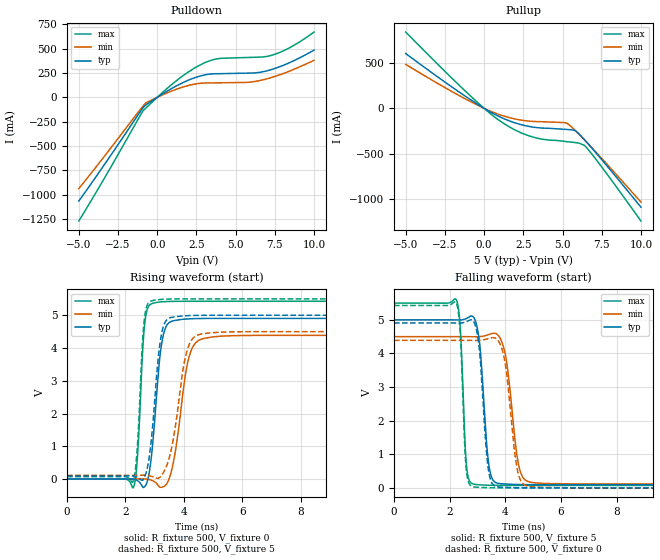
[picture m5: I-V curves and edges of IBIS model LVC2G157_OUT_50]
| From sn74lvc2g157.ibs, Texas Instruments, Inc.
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[Model]   LVC2G157_OUT_50
Model_type  Output
Vref =   0
Rref =   500
Cref =   50p
Vmeas =   2.5
| variable   typ   min   max
C_comp   8.88pF   5.48pF   12.17pF
| C_pullup   9.50pF   5.48pF   12.17pF
| C_pulldown   8.25pF   6.13pF   11.11pF
[Temperature Range]   40   100   -40
| Ambient temperature   25   85   -40
[Voltage range]   5   4.5   5.5
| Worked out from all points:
|   slope of the pulldown table from 0 to 0.75 V, typ, clamps not added: 9.95 ohm
|   slope of the pullup table from 0 to 0.75 V, typ, clamps not added: 10.3 ohm
|   rising waveform, R_fixture 500, V_fixture 0: 20-80 % time 283ps typ, 407ps min, 181ps max; typ from 0 V to 4.9 V
|   falling waveform, R_fixture 500, V_fixture 5: 20-80 % time 245ps typ, 345ps min, 159ps max; typ from 5 V to 0.093 V
|   rising waveform, R_fixture 500, V_fixture 5: 20-80 % time 293ps typ, 440ps min, 182ps max; typ from 0.093 V to 5 V
|   falling waveform, R_fixture 500, V_fixture 0: 20-80 % time 242ps typ, 334ps min, 155ps max; typ from 4.91 V to 0 V
[Pulldown]
| LVC2G157_OUT_50
|   Voltage   I(typ)   I(min)   I(max)
-5V       -1.064A    -937.1mA   -1.27A
-3.355V   -687.5mA   -602.1mA   -826.3mA
-925mV    -111.5mA   -92.93mA   -143.7mA
-620mV    -65.83mA   -48.5mA    -93.56mA
1.13V     109.8mA    78.31mA    159.2mA
2.415V    202.9mA    136.7mA    304.4mA
3.52V     241.4mA    148.6mA    384.4mA
5.67V     248.7mA    153.7mA    409.3mA
6.55V     257.8mA    173.2mA    413.7mA
7.245V    283.9mA    202mA      430mA
8.045V    329.6mA    245.5mA    478mA
10V       485.6mA    380.4mA    671.3mA
[Pullup]
| LVC2G157_OUT_50
|   Voltage   I(typ)   I(min)   I(max)
-5V       604.5mA    484.9mA    841.8mA
-1.075V   119.7mA    93.33mA    170.1mA
205mV     -21.37mA   -16.3mA    -30.84mA
1.085V    -100.6mA   -75.34mA   -147.2mA
2.055V    -164.7mA   -120mA     -245.4mA
3.025V    -204.3mA   -143.2mA   -312mA
3.86V     -218.8mA   -148.7mA   -344.2mA
5.29V     -233.1mA   -166mA     -367.5mA
5.825V    -248.5mA   -246.2mA   -378.1mA
6.49V     -363.8mA   -364.1mA   -425.3mA
7.725V    -612.1mA   -595.3mA   -698.9mA
10V       -1.09A     -1.034A    -1.243A
[Ramp]
| LVC2G157_OUT_50
| variable   typ   min   max
dV/dt_r   3.10/3.12E-10   2.78/4.40E-10   3.42/1.94E-10
dV/dt_f   3.01/2.60E-10   2.69/3.61E-10   3.33/1.65E-10
R_load = 500
[Rising Waveform]
| LVC2G157_OUT_50
R_fixture =   500
C_fixture =   0
L_fixture =   0
V_fixture =   0
V_fixture_min = 0
V_fixture_max = 0
|   Time   V(typ)   V(min)   V(max)
0s        187.4pV    4.471nV    591.1pV
2.275ns   -2.539mV   258.5uV    -248.9mV
2.41ns    -46.69mV   1.381mV    678.3mV
2.66ns    -227.1mV   4.361mV    4.753V
2.965ns   1.407V     -67.03mV   5.372V
3.18ns    3.746V     -247.6mV   5.404V
3.385ns   4.647V     -175.4mV   5.418V
4.175ns   4.89V      3.718V     5.426V
4.715ns   4.902V     4.299V     5.427V
24.99ns   4.904V     4.387V     5.427V
[Falling Waveform]
| LVC2G157_OUT_50
R_fixture =   500
C_fixture =   0
L_fixture =   0
V_fixture =   5
V_fixture_min = 4.5
V_fixture_max = 5.5
|   Time   V(typ)   V(min)   V(max)
0s        5V         4.5V       5.5V
2.245ns   4.999V     4.5V       5.592V
2.385ns   4.998V     4.5V       4.723V
2.605ns   5.043V     4.5V       665.4mV
2.85ns    5.089V     4.498V     112.2mV
3.415ns   644.2mV    4.565V     77.83mV
3.725ns   136.2mV    4.556V     74.26mV
4.48ns    99.06mV    667.1mV    72.31mV
4.87ns    95.22mV    172.5mV    72.13mV
24.99ns   92.94mV    113.9mV    72.02mV
[Rising Waveform]
| LVC2G157_OUT_50
R_fixture =   500
C_fixture =   0
L_fixture =   0
V_fixture =   5
V_fixture_min = 4.5
V_fixture_max = 5.5
|   Time   V(typ)   V(min)   V(max)
0s        92.92mV    113.9mV    72.01mV
2.255ns   93.02mV    114mV      -85.97mV
2.4ns     57.17mV    115.1mV    908.6mV
2.64ns    38.69mV    118.5mV    4.821V
2.95ns    1.828V     66.68mV    5.451V
3.15ns    3.931V     37.76mV    5.478V
3.33ns    4.735V     250mV      5.49V
4.09ns    4.986V     3.861V     5.5V
4.585ns   4.997V     4.425V     5.5V
24.99ns   5V         4.5V       5.5V
[Falling Waveform]
| LVC2G157_OUT_50
R_fixture =   500
C_fixture =   0
L_fixture =   0
V_fixture =   0
V_fixture_min = 0
V_fixture_max = 0
|   Time   V(typ)   V(min)   V(max)
0s        4.907V     4.391V     5.429V
2.245ns   4.906V     4.391V     5.495V
2.38ns    4.905V     4.391V     4.606V
2.59ns    4.942V     4.391V     610.3mV
2.845ns   4.971V     4.389V     30.29mV
3.065ns   4.133V     4.392V     14.74mV
3.385ns   574mV      4.44V      5.278mV
3.675ns   36.74mV    4.439V     2.179mV
4.785ns   2.047mV    51.21mV    133.9uV
24.99ns   15.26uV    23.65uV    11.15uV
